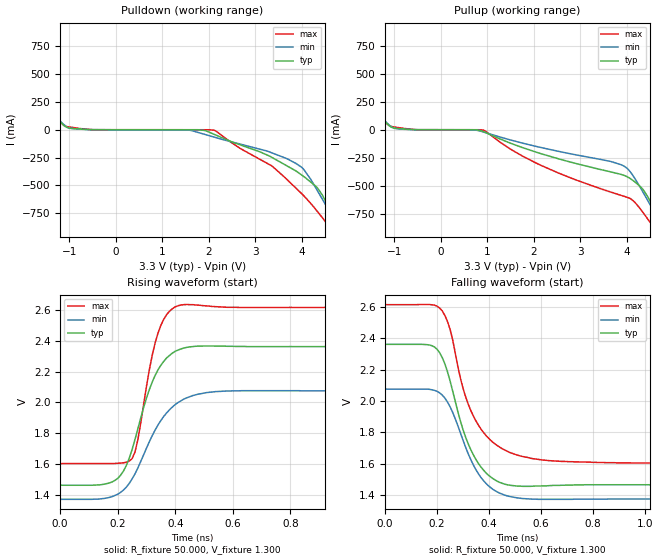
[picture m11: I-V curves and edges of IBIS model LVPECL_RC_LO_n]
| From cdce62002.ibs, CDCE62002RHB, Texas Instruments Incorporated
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|   Model LVPECL_RC_LO_n LVPECL LO SWING for UXN Pins
[Model]   LVPECL_RC_LO_n
Model_type   Output_ECL
Polarity   Non-Inverting
Enable   Active-High
Vmeas = 1.5
Vref = 0
Cref = 0
Rref = 150
|   typ   min   max
|   Strong PVT   Nominal PVT  Weak PVT
C_comp   1.8497pF   1.8465pF   1.8619pF
[Voltage Range]   3.3   3   3.6
[Temperature Range]   40   100   -40
[Pullup Reference]   3.3   3   3.6
[Pulldown Reference]   3.3   3   3.6
[Power Clamp Reference]   3.3   3   3.6
[GND Clamp Reference]   0   0   0
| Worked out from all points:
|   falling waveform, R_fixture 50.000, V_fixture 1.300: 20-80 % time 103ps typ, 110ps min, 118ps max; typ from 2.36 V to 1.47 V
|   rising waveform, R_fixture 50.000, V_fixture 1.300: 20-80 % time 91.1ps typ, 118ps min, 59.9ps max; typ from 1.47 V to 2.36 V
[Pulldown]
|   Voltage   I(typ)   I(min)   I(max)
-3.3V     1.332A     1.268A     1.424A
-2.68V    935.4mA    899.2mA    1.004A
-1.288V   115mA      119.3mA    116.2mA
-1.042V   18.84mA    20.53mA    27.56mA
1.586V    -109.5uA   -4.153mA   -17.03uA
2.111V    -40.58mA   -65.67mA   -4.131mA
3.352V    -247mA     -206.9mA   -324.1mA
3.992V    -405.1mA   -335.5mA   -571.5mA
4.342V    -525.1mA   -551.5mA   -737.5mA
4.689V    -781.1mA   -805.6mA   -932mA
4.89V     -953.1mA   -957.8mA   -1.114A
6.6V      -2.418A    -2.277A    -2.862A
[Pullup]
|   Voltage   I(typ)   I(min)   I(max)
-3.3V     1.332A     1.269A     1.435A
-2.63V    904.6mA    868.5mA    966.5mA
-1.29V    115.3mA    120.4mA    117.6mA
-1.067V   23.18mA    26.86mA    29.91mA
918mV     -17.48mA   -20.67mA   -4.542mA
2.059V    -201.7mA   -150.1mA   -300mA
3.672V    -378.5mA   -285.8mA   -559.7mA
4.02V     -422.7mA   -350mA     -605.8mA
4.317V    -519.2mA   -535mA     -722.3mA
4.665V    -763.2mA   -788.8mA   -915mA
4.838V    -904.1mA   -917.4mA   -1.054A
6.6V      -2.409A    -2.271A    -2.848A
[Ramp]
R_load = 50
|   typ   min   max
dV/dt_r   0.557474/9.11089e-11   0.420555/1.18172e-10   0.60585/5.99348e-11
dV/dt_f   0.557443/1.02798e-10   0.420514/1.09971e-10   0.60586/1.18597e-10
[Falling Waveform]
R_fixture = 50.000
V_fixture = 1.300
V_fixture_min = 1.000
V_fixture_max = 1.600
C_fixture = 0.000
|  time   V(typ)   V(min)   V(max)
0s        2.361V     2.075V     2.614V
170ps     2.357V     2.074V     2.615V
220ps     2.276V     2.037V     2.574V
250ps     2.128V     1.963V     2.457V
300ps     1.816V     1.749V     2.08V
340ps     1.655V     1.59V      1.903V
410ps     1.51V      1.442V     1.743V
500ps     1.458V     1.384V     1.659V
750ps     1.464V     1.373V     1.61V
1.7ns     1.465V     1.374V     1.605V
[Rising Waveform]
R_fixture = 50.000
V_fixture = 1.300
V_fixture_min = 1.000
V_fixture_max = 1.600
C_fixture = 0.000
|  time   V(typ)   V(min)   V(max)
0s        1.465V     1.374V     1.605V
180ps     1.486V     1.391V     1.605V
220ps     1.557V     1.434V     1.61V
250ps     1.696V     1.506V     1.637V
270ps     1.83V      1.577V     1.76V
310ps     2.084V     1.747V     2.213V
340ps     2.211V     1.855V     2.449V
410ps     2.339V     2V         2.625V
580ps     2.363V     2.074V     2.615V
1.7ns     2.361V     2.075V     2.614V
